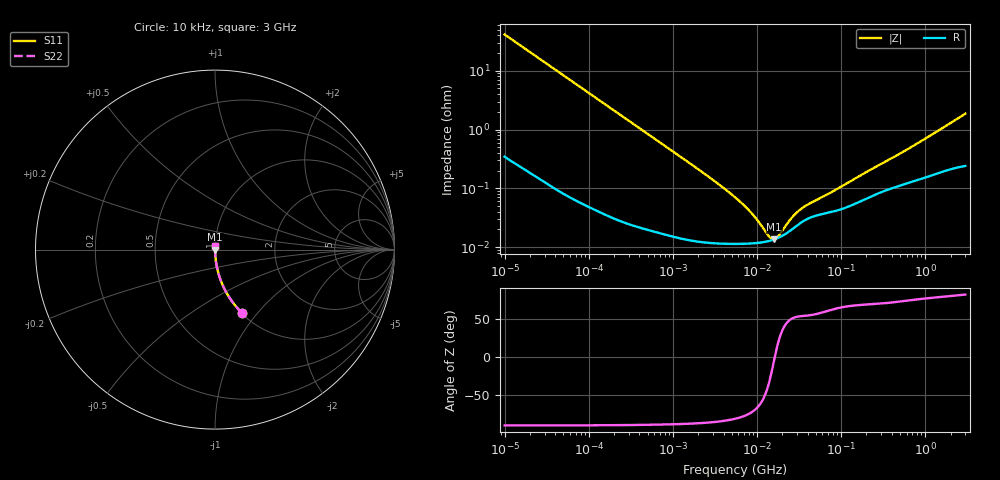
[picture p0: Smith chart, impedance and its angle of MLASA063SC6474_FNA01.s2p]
! MLASA063SC6474_FNA01  S-PARAMETER MODEL  ( Standard Model )
! Model Generated by TAIYO YUDEN Corporation (http://www.ty-top.com)
! Version 2.0
! TAIYO YUDEN Control No. 240306
! Copyright(c) 2013 TAIYO YUDEN CO.,LTD. All Rights Reserved.
! Product Description (link to TY-COMPAS)
! https://ds.yuden.co.jp/TYCOMPAS/or/detail?pn=MLASA063SC6474KFNA01&u=M
! Products Name : Multilayer Ceramic Capacitors
! Characteristics :
!  Capacitance : 0.47 [uF] , Rated Voltage : 4 [V] , TCC : X6S
!  Case Size : 0.6 x 0.3 / 0.024 x 0.012 [mm/inch] , Thickness : 0.3 / 0.012 [mm/inch]
!  (Conditions: Temperature = 25 [degC] , DC Bias Voltage = 0 [V])
! External Node Assignments :
!  1  o---| |---o  2
! GND o---------o GND
! Frequency Range : 10kHz  -  3GHz  [ 401 STEP ]
# MHZ S RI R 50
! Freq[MHz].  S11 Real  S11 Imag  S21 Real  S21 Imag  S12 Real  S12 Imag  S22 Real  S22 Imag
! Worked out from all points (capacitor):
!   401 points, 10 kHz to 3 GHz, reference 50 ohm
!   read as one part in series: C = 383 nF near 10.65 kHz
!   lowest |Z| = 13.5 mohm at 16 MHz (marker M1)
!   series resonance near 16.24 MHz, so ESL is about 250 pH
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0.01  0.1489 -0.3519  0.8511 0.3519  0.8511 0.3519  0.1489 -0.3519
0.016047  0.0648 -0.2418  0.9352 0.2418  0.9352 0.2418  0.0648 -0.2418
0.027426  0.0239 -0.1482  0.9761 0.1482  0.9761 0.1482  0.0239 -0.1482
0.045421  0.00926 -0.0911  0.9907 0.0911  0.9907 0.0911  0.00926 -0.0911
0.082683  0.00311 -0.0505  0.9969 0.0505  0.9969 0.0505  0.00311 -0.0505
0.199902  0.000749 -0.0211  0.9993 0.0211  0.9993 0.0211  0.000749 -0.0211
0.683653  0.000212 -0.00621  0.9998 0.00621  0.9998 0.00621  0.000212 -0.00621
2.652321  0.00012 -0.00157  0.9999 0.00157  0.9999 0.00157  0.00012 -0.00157
5.477226  0.000114 -0.000697  0.9999 0.000697  0.9999 0.000697  0.000114 -0.000697
8.789267  0.000116 -0.000348  0.9999 0.000348  0.9999 0.000348  0.000116 -0.000348
14.10408  0.000128 -7.57e-05  0.9999 7.57e-05  0.9999 7.57e-05  0.000128 -7.57e-05
15.02209  0.000131 -4.17e-05  0.9999 4.17e-05  0.9999 4.17e-05  0.000131 -4.17e-05
15.99985  0.000135 -8.02e-06  0.9999 8.02e-06  0.9999 8.02e-06  0.000135 -8.02e-06
18.15044  0.000145 5.92e-05  0.9999 -5.92e-05  0.9999 -5.92e-05  0.000145 5.92e-05
24.10585  0.000184 0.000208  0.9998 -0.000208  0.9998 -0.000208  0.000184 0.000208
29.12589  0.000226 0.000301  0.9998 -0.000301  0.9998 -0.000301  0.000226 0.000301
35.19136  0.000274 0.000383  0.9997 -0.000383  0.9997 -0.000383  0.000274 0.000383
45.28751  0.000327 0.000481  0.9997 -0.000481  0.9997 -0.000481  0.000327 0.000481
75.00035  0.000393 0.000746  0.9996 -0.000746  0.9996 -0.000746  0.000393 0.000746
374.4521  0.000976 0.00293  0.999 -0.00293  0.999 -0.00293  0.000976 0.00293
749.2693  0.00136 0.00528  0.9986 -0.00528  0.9986 -0.00528  0.00136 0.00528
3000  0.00274 0.0184  0.9973 -0.0184  0.9973 -0.0184  0.00274 0.0184
